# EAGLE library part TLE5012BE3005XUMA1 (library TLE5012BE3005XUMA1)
INFINEON - TLE5012BE3005XUMA1 - GMR Angle Sensor, 3V to 5.5V, SOIC-8 Source: Datasheet
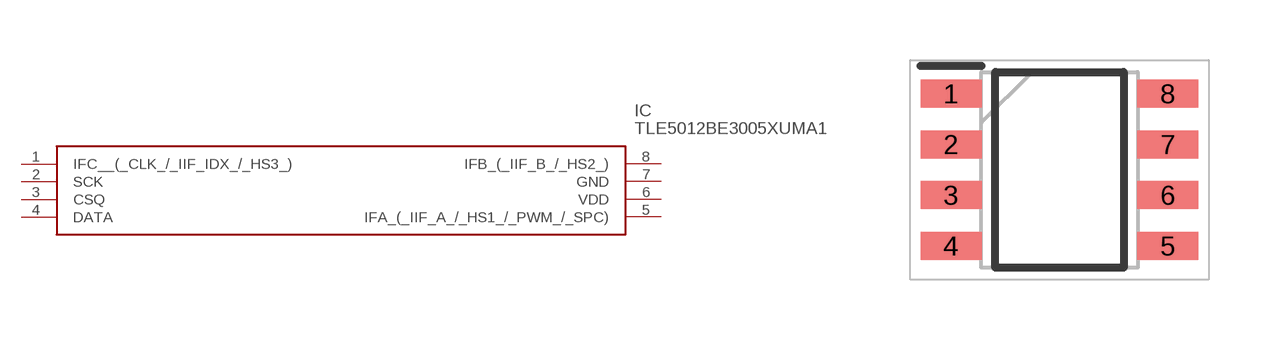
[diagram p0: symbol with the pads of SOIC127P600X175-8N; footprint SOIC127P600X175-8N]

Designator prefix IC

## TLE5012BE3005XUMA1 (Arrow_Part_Number: TLE5012BE3005XUMA1; Arrow_Price-Stock: https://www.arrow.com/en/products/tle5012be3005xuma1/infineon-technologies-ag?utm_currency=USD&region=nac; Description: INFINEON - TLE5012BE3005XUMA1 - GMR Angle Sensor, 3V to 5.5V, SOIC-8; Height: 1.75mm; Manufacturer_Name: Infineon; Manufacturer_Part_Number: TLE5012BE3005XUMA1; Mouser_Part_Number: 726-TLE5012BE3005X; Mouser_Price-Stock: https://www.mouser.co.uk/ProductDetail/Infineon-Technologies/TLE5012BE3005XUMA1?qs=3Bi3m9r5MQbrmq0P2z8x%252Bg%3D%3D)  [SOIC127P600X175-8N]
1  IFC__(_CLK_/_IIF_IDX_/_HS3_)
2  SCK  in
3  CSQ  in
4  DATA
5  IFA_(_IIF_A_/_HS1_/_PWM_/_SPC)
6  VDD  pwr
7  GND  pwr
8  IFB_(_IIF_B_/_HS2_)  out

## Footprint SOIC127P600X175-8N (pad centres in mm)
TLE5012B E3005
smd 1.525 x 0.7: 1 -2.712,1.905; 2 -2.712,0.635; 3 -2.712,-0.635; 4 -2.712,-1.905; 5 2.712,-1.905; 6 2.712,-0.635; 7 2.712,0.635; 8 2.712,1.905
